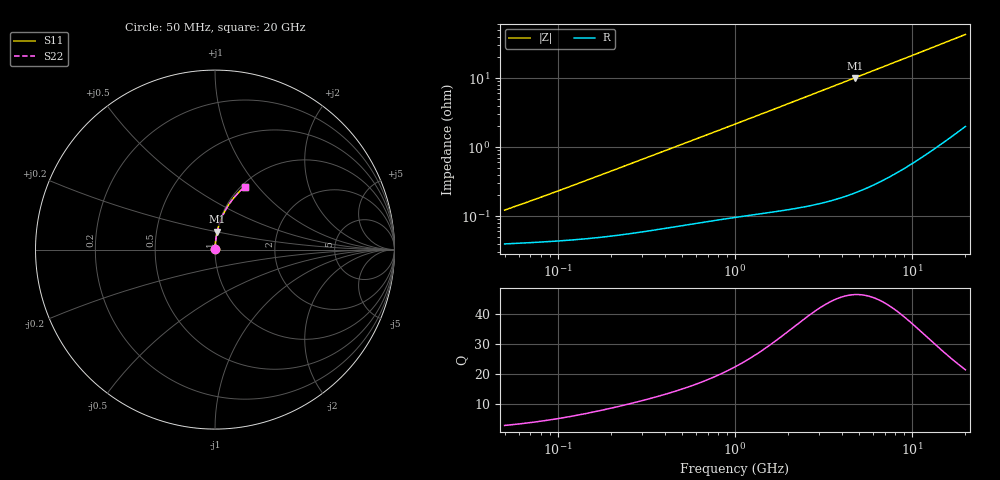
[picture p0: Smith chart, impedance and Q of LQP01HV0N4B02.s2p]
!Murata Part Number: LQP01HV0N4B02
!These Parameters are Measured in Series Mode Connection
!  o--[Z]--o
!Port1  Port2
!  o-------o
!Freq. Start=50[MHz] Stop=20[GHz], 401[Steps]
# Hz S RI R 50
!Freq.(Hz) S11(Real) S11(Imag) S21(Real) S21(Imag) S12(Real) S12(Imag) S22(Real) S22(Imag)
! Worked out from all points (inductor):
!   401 points, 50 MHz to 20 GHz, reference 50 ohm
!   read as one part in series: L = 366 pH near 51.52 MHz
!   highest Q = 46.6 at 4.748 GHz (marker M1), where L = 338 pH
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5e7  0.000397 0.00116  0.9996 -0.00116  0.9996 -0.00116  0.000397 0.00116
5.152053e7  0.000398 0.00119  0.9996 -0.00119  0.9996 -0.00119  0.000398 0.00119
7.162978e7  0.000417 0.00164  0.9996 -0.00164  0.9996 -0.00164  0.000417 0.00164
9.664883e7  0.000438 0.0022  0.9996 -0.0022  0.9996 -0.0022  0.000438 0.0022
1.364002e8  0.000473 0.00308  0.9995 -0.00308  0.9995 -0.00308  0.000473 0.00308
3.721004e8  0.00071 0.00819  0.9993 -0.00819  0.9993 -0.00819  0.00071 0.00819
6.380365e8  0.000995 0.0138  0.999 -0.0138  0.999 -0.0138  0.000995 0.0138
1e9  0.00142 0.0215  0.9986 -0.0215  0.9986 -0.0215  0.00142 0.0215
1.714689e9  0.0025 0.0365  0.9975 -0.0365  0.9975 -0.0365  0.0025 0.0365
2.728004e9  0.00478 0.0577  0.9952 -0.0577  0.9952 -0.0577  0.00478 0.0577
3.626126e9  0.0076 0.0764  0.9924 -0.0764  0.9924 -0.0764  0.0076 0.0764
4.748272e9  0.0122 0.0995  0.9878 -0.0995  0.9878 -0.0995  0.0122 0.0995
5.944466e9  0.0183 0.1237  0.9817 -0.1237  0.9817 -0.1237  0.0183 0.1237
7.442007e9  0.0278 0.1533  0.9722 -0.1533  0.9722 -0.1533  0.0278 0.1533
9.892087e9  0.0474 0.1994  0.9526 -0.1994  0.9526 -0.1994  0.0474 0.1994
1.131968e10  0.0608 0.2248  0.9392 -0.2248  0.9392 -0.2248  0.0608 0.2248
1.276073e10  0.0758 0.2492  0.9242 -0.2492  0.9242 -0.2492  0.0758 0.2492
1.417136e10  0.0917 0.2718  0.9083 -0.2718  0.9083 -0.2718  0.0917 0.2718
1.573793e10  0.1106 0.2953  0.8894 -0.2953  0.8894 -0.2953  0.1106 0.2953
1.747767e10  0.1328 0.3194  0.8672 -0.3194  0.8672 -0.3194  0.1328 0.3194
1.940974e10  0.1588 0.3436  0.8412 -0.3436  0.8412 -0.3436  0.1588 0.3436
2e10  0.167 0.3504  0.833 -0.3504  0.833 -0.3504  0.167 0.3504
